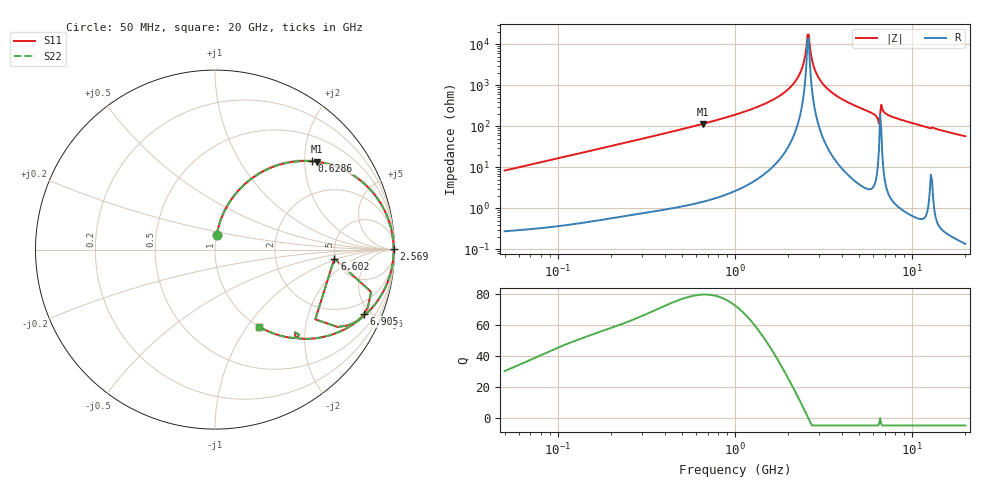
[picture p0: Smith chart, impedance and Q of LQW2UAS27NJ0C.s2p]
!Murata Part Number: LQW2UAS27NJ0C
!These Parameters are Measured in Series Mode Connection
!  o--[Z]--o
!Port1  Port2
!  o-------o
!Freq. Start=50[MHz] Stop=20[GHz], 401[Steps]
# Hz S RI R 50
!Freq.(Hz) S11(Real) S11(Imag) S21(Real) S21(Imag) S12(Real) S12(Imag) S22(Real) S22(Imag)
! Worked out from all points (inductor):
!   401 points, 50 MHz to 20 GHz, reference 50 ohm
!   read as one part in series: L = 26.4 nH near 51.52 MHz
!   highest Q = 79.8 at 657.4 MHz (marker M1), where L = 27.7 nH
!   self-resonance near 2.569 GHz
!   S11 on the Smith chart (normalised r, x): 50 MHz: 1.01, +0.17; 628.6 MHz: 1.03, +2.18; 2.569 GHz: open; 6.602 GHz: 4.84, -0.87; 6.905 GHz: 1.16, -4.56; 20 GHz: 1.00, -1.14
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5e7  0.00953 0.082  0.9905 -0.082  0.9905 -0.082  0.00953 0.082
1.364002e8  0.052 0.2125  0.948 -0.2125  0.948 -0.2125  0.052 0.2125
3.721004e8  0.2807 0.4424  0.7193 -0.4424  0.7193 -0.4424  0.2807 0.4424
6.285508e8  0.5415 0.492  0.4585 -0.492  0.4585 -0.492  0.5415 0.492
6.574395e8  0.5662 0.4894  0.4338 -0.4894  0.4338 -0.4894  0.5662 0.4894
1e9  0.7819 0.4061  0.2181 -0.4061  0.2181 -0.4061  0.7819 0.4061
1.544007e9  0.9337 0.2385  0.0663 -0.2385  0.0663 -0.2385  0.9337 0.2385
2.021818e9  0.9814 0.1161  0.0186 -0.1161  0.0186 -0.1161  0.9814 0.1161
2.348516e9  0.9932 0.046  0.00679 -0.046  0.00679 -0.046  0.9932 0.046
2.569357e9  0.9954 0.00363  0.00458 -0.00363  0.00458 -0.00363  0.9954 0.00363
2.647493e9  0.9953 -0.0105  0.00466 0.0105  0.00466 0.0105  0.9953 -0.0105
2.728004e9  0.9949 -0.0247  0.00513 0.0247  0.00513 0.0247  0.9949 -0.0247
2.810964e9  0.994 -0.0388  0.00602 0.0388  0.00602 0.0388  0.994 -0.0388
2.98453e9  0.991 -0.0672  0.00901 0.0672  0.00901 0.0672  0.991 -0.0672
3.572216e9  0.9719 -0.1517  0.0281 0.1517  0.0281 0.1517  0.9719 -0.1517
6.217679e9  0.7645 -0.4122  0.2355 0.4122  0.2355 0.4122  0.7645 -0.4122
6.406762e9  0.6836 -0.4312  0.3164 0.4312  0.3164 0.4312  0.6836 -0.4312
6.601595e9  0.6649 -0.0498  0.3351 0.0498  0.3351 0.0498  0.6649 -0.0498
6.905011e9  0.83 -0.3583  0.17 0.3583  0.17 0.3583  0.83 -0.3583
7.442007e9  0.7654 -0.4183  0.2346 0.4183  0.2346 0.4183  0.7654 -0.4183
1.131968e10  0.5187 -0.497  0.4813 0.497  0.4813 0.497  0.5187 -0.497
2e10  0.2445 -0.4286  0.7555 0.4286  0.7555 0.4286  0.2445 -0.4286
